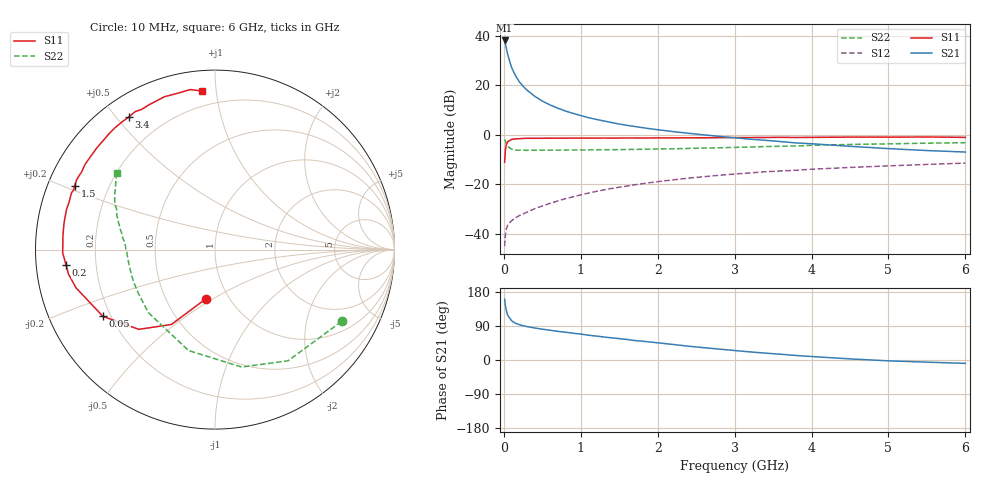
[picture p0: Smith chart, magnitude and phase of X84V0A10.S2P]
! SIEMENS Small Signal Semiconductors
! BFP136W
! Si NPN RF Bipolar Junction Transistor in SOT343
! VCE = 4 V  IC = 100 mA
! Common Emitter S-Parameters:  September  1994
# GHz  S  MA  R  50
!  f  S11  S21  S12  S22
! GHz  MAG  ANG  MAG  ANG  MAG  ANG  MAG  ANG
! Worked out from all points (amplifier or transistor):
!   40 points, 10 MHz to 6 GHz, reference 50 ohm
!   highest |S21| = 38.1 dB at 10 MHz (marker M1)
!   |S21| within 3 dB of that: start of sweep to 31.43 MHz
!   unconditionally stable (mu >= 1): 571.3 MHz to 2.965 GHz
!   at 200 MHz: K = 0.67, MSG = 27.1 dB, |S12| = -32.7 dB
!   at 1.5 GHz: K = 1.10, MAG = 10.8 dB, |S12| = -21.2 dB
!   at 6 GHz: K = 0.97, MSG = 2.2 dB, |S12| = -11.4 dB
!   S11 on the Smith chart (normalised r, x): 10 MHz: 0.78, -0.46; 50 MHz: 0.17, -0.27; 200 MHz: 0.09, -0.05; 1.5 GHz: 0.08, +0.22; 3.4 GHz: 0.08, +0.54; 6 GHz: 0.11, +0.92
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0.01  0.2784 -100.5  80.7 160.4  0.0056 67.7  0.8107 -29.6
0.02  0.4829 -120.2  69.27 144.0  0.0094 58.5  0.7412 -56.7
0.03  0.6145 -133.7  58.51 132.3  0.0121 50.3  0.671 -77.2
0.05  0.7267 -149.2  41.86 118.2  0.0149 40.4  0.5814 -104.7
0.1  0.8031 -164.6  23.15 103.7  0.0183 37.0  0.5111 -136.7
0.15  0.8276 -170.5  15.77 97.2  0.0209 39.6  0.4917 -150.1
0.2  0.8345 -174.1  11.86 93.3  0.0232 41.4  0.4881 -157.4
0.25  0.8427 -177.1  9.573 90.5  0.0252 43.8  0.4867 -162.0
0.3  0.849 -178.7  8.001 88.3  0.0272 46.1  0.4853 -165.2
0.4  0.8485 177.3  6.03 84.4  0.032 49.9  0.4861 -169.5
0.5  0.8505 174.8  4.807 81.3  0.0363 53.2  0.4871 -172.3
0.6  0.8516 172.7  4.012 78.7  0.0411 55.0  0.4879 -174.2
0.7  0.8537 170.2  3.461 75.6  0.046 56.9  0.4892 -175.6
0.9  0.8555 166.5  2.709 70.7  0.0557 58.8  0.4914 -178.3
1.1  0.8549 162.1  2.215 65.4  0.0662 59.6  0.4949 -180.0
1.5  0.8587 155.5  1.651 56.4  0.0871 59.2  0.5014 176.9
2.2  0.8656 143.2  1.159 41.0  0.1227 54.6  0.5211 171.5
3.2  0.8798 126.3  0.816 21.4  0.1694 45.5  0.5655 162.8
3.4  0.8815 123.1  0.773 18.1  0.179 43.4  0.5783 161.0
4.5  0.897 108.3  0.585 2.9  0.2187 33.4  0.637 151.4
5.5  0.9024 98.8  0.48 -5.7  0.2515 25.7  0.6771 144.7
6  0.886 94.6  0.448 -8.9  0.2677 21.3  0.6927 141.8
